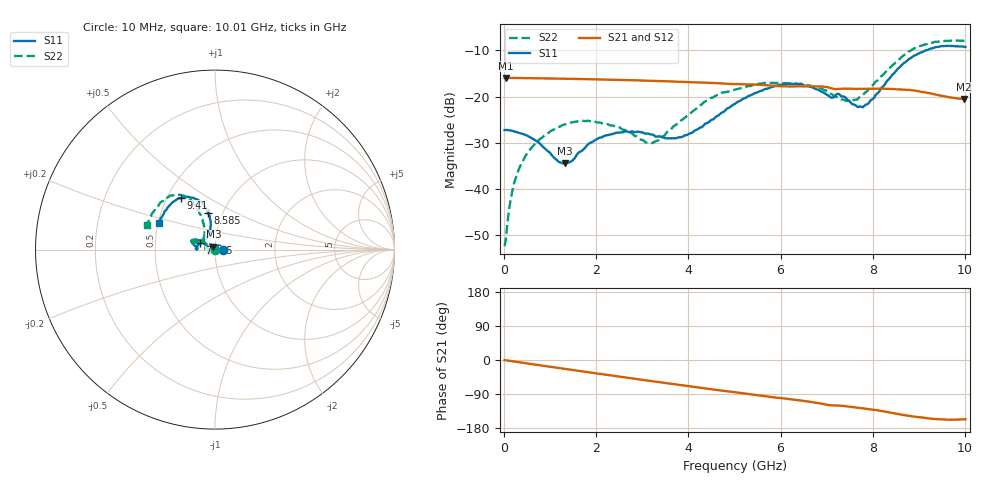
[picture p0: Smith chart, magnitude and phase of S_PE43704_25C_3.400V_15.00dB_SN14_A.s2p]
! Device ID: PE43704
! Dir: z:\PE43704\PE43704_Char_1_20130516\PE43704\AMB\3p400V\15p00dB
! Serial: 14
! Insertion: A
! Impedance: 50 ohm
! Temp: Amb
! VDD: 3.400V
! Attenuation Step: 15.00dB
! IDD: 1.139463e-01mA
#  Hz  S  RI  R  50
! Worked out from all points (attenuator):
!   401 points, 10 MHz to 10.01 GHz, reference 50 ohm
!   highest |S21| = -15.94 dB at 35 MHz (marker M1); lowest = -20.5 dB at 9.985 GHz (marker M2)
!   lowest |S11| = -34.5 dB at 1.31 GHz (marker M3), VSWR 1.04, Z = 49.1 + j1.64 ohm
!   |S11| at or under -10 dB: start of sweep to 9.152 GHz
!   |S22| runs from -52.3 to -7.8 dB; largest |S21 - S12| = 0.0012
!   S11 on the Smith chart (normalised r, x): 10 MHz: 1.09, +0.00; 7.485 GHz: 0.84, +0.06; 8.585 GHz: 0.85, +0.36; 9.41 GHz: 0.59, +0.38; 10.01 GHz: 0.51, +0.17
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1e7  0.0435 0.00025  0.1597 -0.000607  0.1597 -0.000547  -0.00236 0.000483
3.5e7  0.0436 0.00127  0.1597 -0.00189  0.1596 -0.00192  -0.00208 0.00188
1.85e8  0.0419 0.00729  0.159 -0.00955  0.1589 -0.00957  -0.00255 0.00974
4.1e8  0.0364 0.0153  0.157 -0.0211  0.1571 -0.0206  -0.00669 0.0191
7.6e8  0.0214 0.0233  0.1533 -0.0373  0.1533 -0.0373  -0.0193 0.0283
1.31e9  -0.00886 0.0167  0.1434 -0.0618  0.1434 -0.0617  -0.0439 0.0237
1.685e9  -0.0257 0.00359  0.1344 -0.077  0.1345 -0.0769  -0.0536 0.012
2.435e9  -0.0353 -0.0202  0.1116 -0.103  0.1117 -0.103  -0.0466 -0.00352
3.11e9  -0.0323 -0.0235  0.0871 -0.1206  0.0872 -0.1205  -0.0312 0.00551
3.36e9  -0.0321 -0.0189  0.0771 -0.1254  0.0772 -0.1252  -0.0313 0.0133
4.035e9  -0.0398 0.00466  0.05 -0.1342  0.0502 -0.1342  -0.0544 0.0362
4.46e9  -0.0494 0.0216  0.0329 -0.1374  0.033 -0.1374  -0.0784 0.0546
5.01e9  -0.0722 0.0421  0.0116 -0.1364  0.0116 -0.1365  -0.1071 0.0518
5.96e9  -0.1204 0.0559  -0.0225 -0.1282  -0.0221 -0.1281  -0.1343 0.0396
6.685e9  -0.1225 0.0305  -0.0464 -0.1204  -0.0467 -0.1203  -0.1262 0.0324
7.485e9  -0.0829 0.0347  -0.0671 -0.1017  -0.067 -0.1018  -0.0703 0.0571
7.835e9  -0.0453 0.0671  -0.0756 -0.0953  -0.0757 -0.0953  -0.058 0.0947
8.36e9  -0.0249 0.1546  -0.0906 -0.0806  -0.0902 -0.0808  -0.0775 0.186
8.585e9  -0.0391 0.2036  -0.0957 -0.0715  -0.0952 -0.0718  -0.1021 0.234
9.41e9  -0.1881 0.2873  -0.0953 -0.0419  -0.0954 -0.0417  -0.2637 0.2905
9.985e9  -0.3059 0.1588  -0.0863 -0.0376  -0.0865 -0.0374  -0.3727 0.1444
1.001e10  -0.3108 0.149  -0.0867 -0.0379  -0.087 -0.0381  -0.3766 0.136
